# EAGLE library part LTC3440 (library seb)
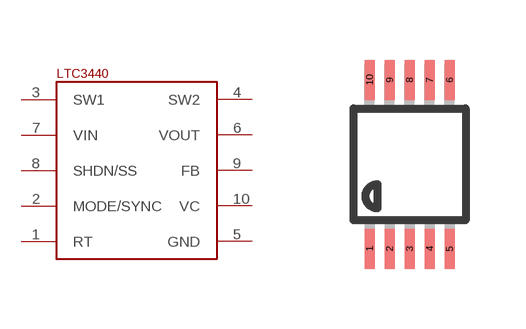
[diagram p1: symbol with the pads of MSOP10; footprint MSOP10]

Designator prefix IC

## LTC3440  [MSOP10]
1  RT
2  MODE/SYNC
3  SW1
4  SW2
5  GND
6  VOUT
7  VIN
8  SHDN/SS
9  FB
10  VC

## Footprint MSOP10 (pad centres in mm)
smd 0.25 x 1: 1 -4.81,-0.843; 2 -4.31,-0.843; 3 -3.81,-0.843; 4 -3.31,-0.843; 5 -2.81,-0.843; 6 -2.81,3.383; 7 -3.31,3.383; 8 -3.81,3.383; 9 -4.31,3.383; 10 -4.81,3.383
